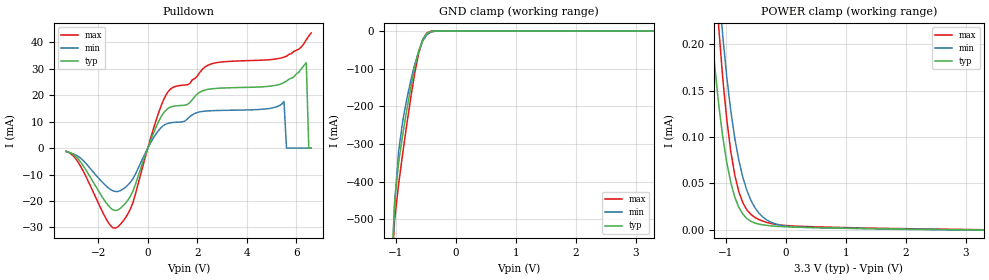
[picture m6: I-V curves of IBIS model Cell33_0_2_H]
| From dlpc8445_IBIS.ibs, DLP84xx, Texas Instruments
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|   Model Cell33_0_2_H
[Model]  Cell33_0_2_H
Model_type I/O_open_drain
Polarity   Non-Inverting
Enable   Active-High
Vinl =  0.990V
Vinh =  2.310V
Vmeas =  1.650V
Cref =  50.000pF
Rref =  1.000M
Vref =  0.0V
C_comp   6.060pF   6.037pF   6.070pF
[Model Spec]
Vinh   2.310V   2.079V   2.541V
Vinl   0.990V   0.891V   1.089V
Vmeas   1.650V   NA   NA
Vref   0.0V   NA   NA
Cref   50.000pF   NA   NA
Rref   1.000M   NA   NA
[Temperature Range]   25.000   0.125k   -40.000
[Voltage Range]   3.300V   2.970V   3.630V
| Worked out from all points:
|   slope of the pulldown table from 0 to 0.495 V, typ, clamps not added: 44.6 ohm
|   GND clamp passes 1 mA (typ) near -0.42 V on its own axis
|   POWER clamp passes 1 mA (typ) near -1.87 V on its own axis
[Pulldown]
|Voltage   I(typ)   I(min)   I(max)
-3.3V     -1.237mA   -1.329mA   -1.147mA
-2.8V     -4.212mA   -3.219mA   -5.536mA
-1.7V     -20.45mA   -14.19mA   -26.45mA
-1.3V     -23.64mA   -16.44mA   -30.29mA
-600mV    -16.25mA   -11.57mA   -20.58mA
700mV     14.06mA    8.936mA    19.5mA
2.3V      21.95mA    13.97mA    30.62mA
5.5V      24.84mA    17.63mA    34.4mA
5.6V      25.35mA    -3.1nA     34.77mA
6.4V      32.3mA     -800nA     40.98mA
6.5V      -100nA     -1.1uA     42.39mA
6.6V      -200nA     -5uA       43.59mA
[GND_clamp]
|Voltage   I(typ)   I(min)   I(max)
-3.3V     -42.11A    -39.21A    -45.03A
-1.089V   -685.9mA   -733.9mA   -690.4mA
-1.022V   -455mA     -457.8mA   -501.3mA
-955mV    -349.5mA   -319.6mA   -406.5mA
-888mV    -276.1mA   -240.2mA   -326.3mA
-821mV    -211.3mA   -182mA     -250.5mA
-687mV    -96.78mA   -88.79mA   -113mA
-620mV    -52.79mA   -53.16mA   -59.38mA
-553mV    -22.32mA   -26.92mA   -22.84mA
-486mV    -6.226mA   -10.63mA   -5.004mA
-285mV    -10.21uA   -113.8uA   -1.604uA
3.3V      0A         0A         0A
[POWER_clamp]
|Voltage   I(typ)   I(min)   I(max)
-3.266V   6.209A     1.842A     17.02A
-1.256V   225.5uA    393.8uA    359.2uA
-1.122V   134.7uA    261.3uA    217.8uA
-1.055V   100.1uA    208.8uA    163.1uA
-988mV    72.34uA    164.6uA    118.8uA
-921mV    50.97uA    128.1uA    84.4uA
-854mV    35.26uA    98.53uA    58.93uA
-720mV    16.98uA    56.64uA    29.27uA
-586mV    9.341uA    31.96uA    16.77uA
-318mV    4.885uA    10.66uA    8.077uA
17mV      3.368uA    4.058uA    4.711uA
3.3V      0A         0A         270nA
[Ramp]
| variable   typ   min   max
dV/dt_r   0.651/0.102n   0.418/0.146n   0.881/79.070p
dV/dt_f   0.649/4.660n   0.412/6.546n   0.881/3.008n
R_load = 50.000
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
